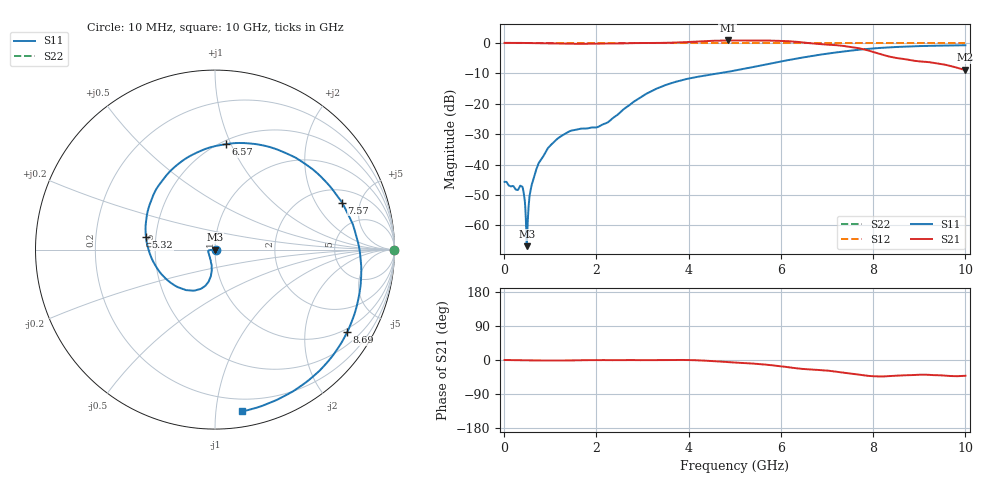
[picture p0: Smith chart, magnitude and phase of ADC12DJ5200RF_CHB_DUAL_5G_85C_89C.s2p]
! Texas Instruments, Inc.
! ADC12DJ5200RF - CH B S-Parameters (Dual Ch Mode, Fs = 5 GSPS, 85 degC case, 89 degC juntion)
! Port 1 represents the 100-ohm differenal input, Port 2 the digital output
! freq  dbS11  angS11  dbS21 angS21 dbS12 angS12 dbS22 angS22
# HZ S DB R 100
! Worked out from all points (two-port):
!   1000 points, 10 MHz to 10 GHz, reference 100 ohm
!   highest |S21| = 0.80 dB at 4.85 GHz (marker M1); lowest = -8.9 dB at 10 GHz (marker M2)
!   |S21| within 3 dB of the highest: start of sweep to 7.821 GHz
!   lowest |S11| = -66.8 dB at 490 MHz (marker M3), VSWR 1.00, Z = 100 + j0.0909 ohm
!   |S11| at or under -10 dB: start of sweep to 4.655 GHz
!   |S22| runs from 0.0 to 0.0 dB; largest |S21 - S12| = 0.77
!   S11 on the Smith chart (normalised r, x): 10 MHz: 1.01, -0.00; 5.32 GHz: 0.44, +0.07; 6.57 GHz: 0.53, +0.96; 7.57 GHz: 2.79, +3.39; 8.69 GHz: 0.87, -3.26; 10 GHz: 0.11, -1.18
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1e7  -45.69 -2.8  0.00 -0.0  0.00 0.0  0.00 0.0
3.8e8  -47.17 -16.4  -0.02 -0.8  0.00 0.0  0.00 0.0
4.9e8  -66.84 93.5  -0.04 -1.0  0.00 0.0  0.00 0.0
5.2e8  -56.15 -177.4  -0.05 -1.1  0.00 0.0  0.00 0.0
5.8e8  -47.93 -158.5  -0.06 -1.2  0.00 0.0  0.00 0.0
6.5e8  -44.16 -162.0  -0.09 -1.2  0.00 0.0  0.00 0.0
9.2e8  -35.36 -172.3  -0.13 -1.3  0.00 0.0  0.00 0.0
1.25e9  -30.53 -174.5  -0.25 -1.4  0.00 0.0  0.00 0.0
1.68e9  -28.19 -167.0  -0.32 -0.5  0.00 0.0  0.00 0.0
2.22e9  -26.31 -127.8  -0.19 -0.3  0.00 0.0  0.00 0.0
3.34e9  -14.84 -101.2  -0.01 -0.3  0.00 0.0  0.00 0.0
4.18e9  -11.19 -124.8  0.45 -0.7  0.00 0.0  0.00 0.0
4.85e9  -9.50 -159.5  0.80 -5.6  0.00 0.0  0.00 0.0
5.01e9  -9.07 -169.7  0.78 -6.8  0.00 0.0  0.00 0.0
5.32e9  -8.17 169.9  0.73 -8.9  0.00 0.0  0.00 0.0
5.9e9  -6.42 130.4  0.70 -15.3  0.00 0.0  0.00 0.0
6.57e9  -4.57 84.1  -0.00 -24.3  0.00 0.0  0.00 0.0
6.67e9  -4.31 77.3  -0.16 -25.3  0.00 0.0  0.00 0.0
7.57e9  -2.45 20.4  -1.44 -37.0  0.00 0.0  0.00 0.0
8.34e9  -1.48 -18.1  -4.46 -42.6  0.00 0.0  0.00 0.0
8.69e9  -1.23 -32.1  -5.36 -40.4  0.00 0.0  0.00 0.0
1e10  -0.78 -80.5  -8.85 -41.7  0.00 0.0  0.00 0.0
